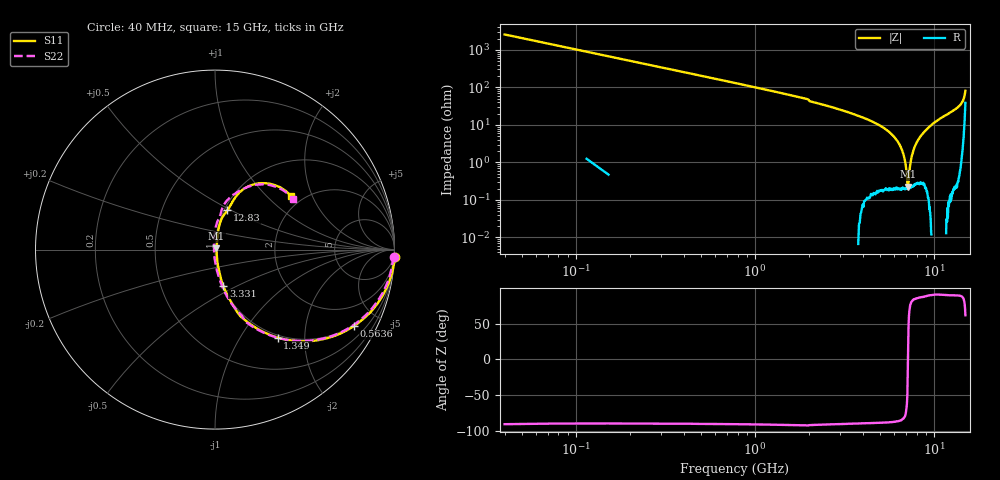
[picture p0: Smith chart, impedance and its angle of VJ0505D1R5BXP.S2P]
! VJ0505D1R5BXP
! MLCC placed on 25 mil thick microstrip substrate in series configuraton.
! DATE 06/29/2018  07:29
! CORRECTED  DATA
# GHz  S  MA  R  50.00
!  FREQ  S11M  S11A  S21M  S21A  S12M  S12A  S22M  S22A
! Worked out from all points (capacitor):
!   401 points, 40 MHz to 15 GHz, reference 50 ohm
!   read as one part in series: C = 1.55 pF near 114.8 MHz
!   lowest |Z| = 226 mohm at 7.146 GHz (marker M1)
!   series resonance near 7.163 GHz, so ESL is about 320 pH
!   S11 on the Smith chart (normalised r, x): 40 MHz: -4, -51; 563.6 MHz: 0.94, -3.65; 1.349 GHz: 0.96, -1.48; 3.331 GHz: 1.01, -0.42; 12.83 GHz: 1.03, +0.48; 15 GHz: 1.74, +1.42
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0.04  1.003 -2.2  0.03885 88.7  0.03973 88.1  0.9954 -2.2
0.227  0.9805 -12.5  0.2166 77.6  0.2167 77.6  0.9724 -12.4
0.5636  0.8829 -28.9  0.4864 61.7  0.486 61.7  0.8759 -29.0
0.9002  0.7563 -42.0  0.6718 49.1  0.672 49.1  0.7519 -42.1
1.349  0.602 -54.5  0.8184 37.1  0.8188 37.1  0.6006 -54.8
2.097  0.3833 -69.8  0.9383 22.8  0.9389 22.8  0.3806 -69.0
2.5458  0.3031 -73.1  0.9595 18.1  0.9598 18.1  0.3048 -73.5
3.3312  0.2055 -77.0  0.9789 12.5  0.9794 12.6  0.2091 -78.7
5.0516  0.08691 -79.5  0.9942 5.7  0.9943 5.7  0.08604 -87.3
6.2484  0.03093 -71.8  0.9967 2.5  0.9973 2.6  0.03021 -98.3
6.585  0.01798 -60.9  0.9972 1.7  0.9977 1.8  0.01719 -107.7
6.959  0.008309 -7.2  0.9972 0.9  0.9978 0.9  0.005588 -162.1
7.0338  0.00845 14.1  0.9973 0.7  0.9975 0.7  0.005541 162.2
7.146  0.01041 36.9  0.9971 0.4  0.9975 0.5  0.007735 131.5
7.52  0.02282 67.9  0.9966 -0.4  0.9971 -0.4  0.0214 103.9
8.3802  0.05416 75.5  0.9948 -2.4  0.995 -2.4  0.05404 95.2
10.0258  0.1172 80.4  0.9925 -6.2  0.9933 -6.2  0.1198 88.5
12.5316  0.2143 74.0  0.9738 -12.5  0.9745 -12.4  0.2222 80.5
12.8308  0.2297 72.6  0.9701 -13.4  0.9702 -13.4  0.2376 79.8
14.3642  0.3582 65.9  0.9179 -21.5  0.9188 -21.5  0.3612 66.6
14.7008  0.4293 58.4  0.855 -25.8  0.855 -25.8  0.4314 57.0
15  0.5192 35.0  0.6419 -27.7  0.6422 -27.6  0.5177 32.7
